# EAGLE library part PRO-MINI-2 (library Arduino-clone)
Arduino Pro Mini Layout 2 Sparkfun.com
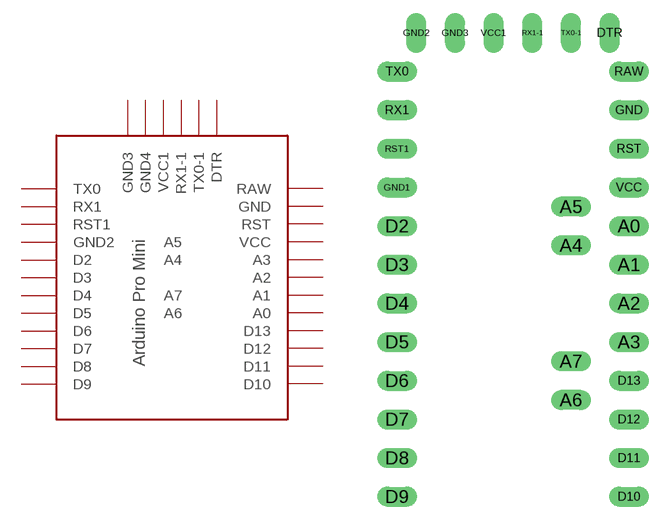
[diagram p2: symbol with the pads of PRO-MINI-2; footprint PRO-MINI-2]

Designator prefix -

## PRO-MINI-2  [PRO-MINI-2]
A0  A0
A1  A1
A2  A2
A3  A3
A4  A4
A5  A5
A6  A6
A7  A7
D2  D2
D3  D3
D4  D4
D5  D5
D6  D6
D7  D7
D8  D8
D9  D9
D10  D10
D11  D11
D12  D12
D13  D13
DTR  DTR
GND  GND
GND1  GND2
GND2  GND3
GND3  GND4
RAW  RAW
RST  RST
RST1  RST1
RX1  RX1
RX1-1  RX1-1
TX0  TX0
TX0-1  TX0-1
VCC  VCC
VCC1  VCC1

## Footprint PRO-MINI-2 (pad centres in mm)
drill 0.8 long: A0 6.35,2.54; A1 6.35,0; A2 6.35,-2.54; A3 6.35,-5.08; A4 2.54,1.27; A5 2.54,3.81; A6 2.54,-8.89; A7 2.54,-6.35; D2 -8.89,2.54; D3 -8.89,0; D4 -8.89,-2.54; D5 -8.89,-5.08; D6 -8.89,-7.62; D7 -8.89,-10.16; D8 -8.89,-12.7; D9 -8.89,-15.24; D10 6.35,-15.24; D11 6.35,-12.7; D12 6.35,-10.16; D13 6.35,-7.62; DTR 5.08,15.24; GND 6.35,10.16; GND1 -8.89,5.08; GND2 -7.62,15.24; GND3 -5.08,15.24; RAW 6.35,12.7; RST 6.35,7.62; RST1 -8.89,7.62; RX1 -8.89,10.16; RX1-1 0,15.24; TX0 -8.89,12.7; TX0-1 2.54,15.24; VCC 6.35,5.08; VCC1 -2.54,15.24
